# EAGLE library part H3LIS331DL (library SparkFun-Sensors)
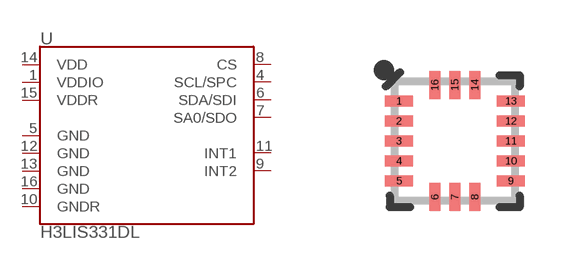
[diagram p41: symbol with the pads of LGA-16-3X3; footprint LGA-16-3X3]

Designator prefix U

## H3LIS331DL (PROD_ID: IC-13786; VALUE: H3LIS331DL)  [LGA-16-3X3]
1  VDDIO
4  SCL/SPC
5  GND
6  SDA/SDI
7  SA0/SDO
8  CS
9  INT2
10  GNDR
11  INT1
12  GND
13  GND
14  VDD
15  VDDR
16  GND

## Footprint LGA-16-3X3 (pad centres in mm)
16-Pin Land Grid Array (LGA) (3 x 3 mm) Datasheet Specifications: Pin Count: 16 Area: 3.0 x 3.0 x 1.0 mm Pitch: 0.5 mm Devices Using: LIS331 LIS3DH
smd 0.7 x 0.28: 1 -1.4,1; 2 -1.4,0.5; 3 -1.4,0; 4 -1.4,-0.5; 5 -1.4,-1; 9 1.4,-1; 10 1.4,-0.5; 11 1.4,0; 12 1.4,0.5; 13 1.4,1
smd 0.28 x 0.7: 6 -0.5,-1.4; 7 0,-1.4; 8 0.5,-1.4; 14 0.5,1.4; 15 0,1.4; 16 -0.5,1.4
